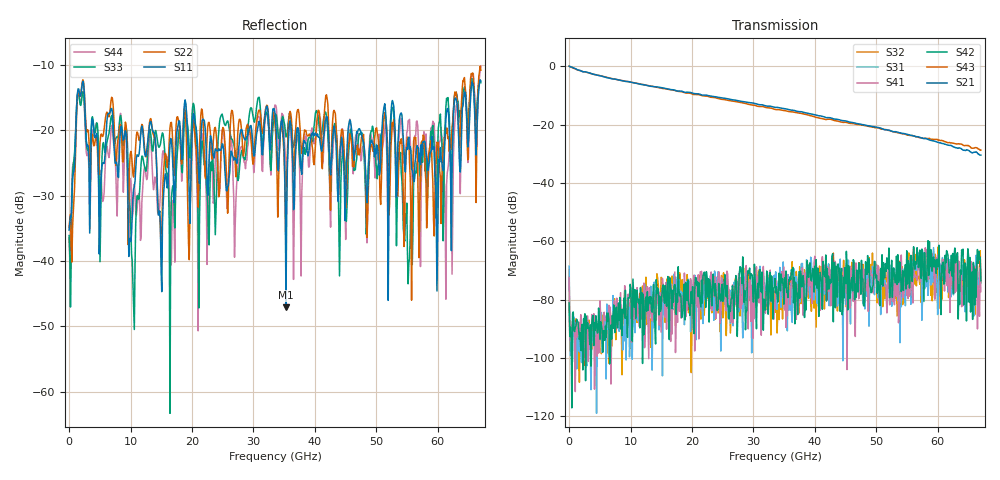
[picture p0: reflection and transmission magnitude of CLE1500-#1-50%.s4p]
!Keysight Technologies,N5247B,US50470101,A.16.20.02
!Date: Thursday, March 13, 2025 10:21:59
!Correction: S11(C  4-Port  )
!S12(C  4-Port  )
!S13(C  4-Port  )
!S14(C  4-Port  )
!S21(C  4-Port  )
!S22(C  4-Port  )
!S23(C  4-Port  )
!S24(C  4-Port  )
!S31(C  4-Port  )
!S32(C  4-Port  )
!S33(C  4-Port  )
!S34(C  4-Port  )
!S41(C  4-Port  )
!S42(C  4-Port  )
!S43(C  4-Port  )
!S44(C  4-Port  )
!S4P File: Measurements: <S11,S12,S13,S14>,
!<S21,S22,S23,S24>,
!<S31,S32,S33,S34>,
!<S41,S42,S43,S44>:
# Hz S  dB  R 50
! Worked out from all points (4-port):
!   601 points, 10 MHz to 67 GHz, reference 50 ohm
!   strongest paths, dB at 10 MHz, 16.76 GHz, 33.51 GHz, 50.25 GHz, 67 GHz:
!     S21: 0.0, -8.0, -14.1, -21.0, -30.5
!     S43: 0.0, -8.1, -14.8, -21.2, -28.8
!     S42: -81.1, -83.1, -72.7, -73.7, -73.5
!     S41: -72.4, -91.8, -83.0, -68.3, -77.2
!     S31: -68.5, -82.4, -73.2, -79.4, -74.5
!     S32: -69.7, -71.9, -84.3, -69.2, -74.1
!   lowest |S11| = -47.1 dB at 35.29 GHz (marker M1), VSWR 1.01, Z = 49.6 - j0.0284 ohm
!   |S11| at or under -10 dB: start of sweep to end of sweep
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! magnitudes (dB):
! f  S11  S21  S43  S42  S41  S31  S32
! 10 MHz  -35.3  0.0  0.0  -81.1  -72.4  -68.5  -69.7
! 1.685 GHz  -14.2  -1.4  -1.5  -93.6  -92.2  -97.9  -108.3
! 10.39 GHz  -30.3  -5.7  -5.6  -73.0  -82.3  -81.8  -80.7
! 13.18 GHz  -18.7  -6.9  -6.8  -81.2  -82.2  -83.9  -87.0
! 35.29 GHz  -47.1  -14.7  -15.3  -70.2  -89.5  -79.4  -83.7
! 55.5 GHz  -22.5  -23.7  -23.8  -69.8  -74.9  -65.4  -70.6
! 67 GHz  -12.4  -30.5  -28.8  -73.5  -77.2  -74.5  -74.1
